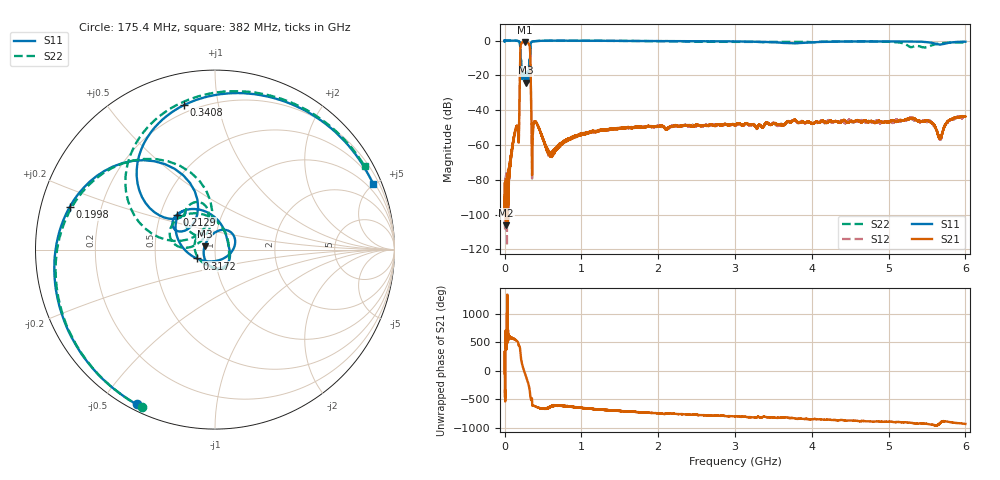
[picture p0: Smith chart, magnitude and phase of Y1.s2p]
!Keysight Technologies,N5232A,MY52221221,A.10.65.11
!Date: Thursday, November 09, 2023 14:39:33
!Correction: S11(Full 2 Port(1,4))
!S41(Full 2 Port(1,4))
!S14(Full 2 Port(1,4))
!S44(Full 2 Port(1,4))
!S2P File: Measurements: S11, S41, S14, S44:
# Hz S  RI  R 50
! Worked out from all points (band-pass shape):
!   16001 points, 300 kHz to 6 GHz, reference 50 ohm
!   highest |S21| = -0.94 dB at 262 MHz (marker M1); lowest = -106.2 dB at 17.92 MHz (marker M2)
!   |S21| within 3 dB of the highest: 206.4 MHz to 329.4 MHz (123 MHz wide, 45.9 % of centre)
!   lowest |S11| = -24.3 dB at 273.3 MHz (marker M3), VSWR 1.13, Z = 44.5 + j1.64 ohm
!   |S11| at or under -10 dB: 206 MHz to 331.9 MHz (125.9 MHz wide, 46.8 % of centre)
!   |S22| runs from -22.2 to 0.0 dB; largest |S21 - S12| = 0.0022
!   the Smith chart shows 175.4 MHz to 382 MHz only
!   S11 on the Smith chart (normalised r, x): 175.4 MHz: 0.02, -0.62; 199.8 MHz: 0.09, +0.14; 212.9 MHz: 0.61, +0.26; 317.2 MHz: 0.81, -0.08; 340.8 MHz: 0.16, +0.80; 382 MHz: 0.61, +4.95
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300000  1.004 -0.00731  5.71e-05 -5.35e-05  3.24e-05 7.01e-06  1.002 -0.0072
1.792412e7  0.9906 -0.133  2.49e-08 4.88e-06  -8.13e-06 -1.72e-05  0.9906 -0.1309
1.086696e8  0.6161 -0.781  -0.000926 -0.00061  -0.000994 -0.000492  0.6305 -0.7709
1.754162e8  -0.4349 -0.8627  -0.00166 0.00147  -0.00174 0.00153  -0.4061 -0.8797
1.9979e8  -0.8096 0.2377  0.0819 0.0818  0.0819 0.0816  -0.7913 0.2473
2.129144e8  -0.2112 0.1954  -0.5439 -0.5433  -0.5434 -0.5435  -0.2351 0.1437
2.305385e8  0.0738 0.0291  -0.2171 0.8498  -0.2173 0.8493  0.0779 0.0046
2.620369e8  -0.0492 -0.068  0.7637 -0.4717  0.7629 -0.4717  0.00628 -0.1071
2.732864e8  -0.0581 0.0184  0.2434 -0.8607  0.2437 -0.86  -0.0247 -0.0936
3.171592e8  -0.1022 -0.0491  -0.00435 0.7967  -0.00382 0.7967  -0.1355 0.0967
3.40783e8  -0.1722 0.8054  -0.0524 -0.0537  -0.0523 -0.0538  -0.3108 0.7425
3.820309e8  0.8809 0.3653  -0.00121 0.00405  -0.00118 0.00411  0.834 0.4635
4.187791e8  0.9697 -0.0672  0.000554 0.00413  0.000571 0.00405  0.9703 0.0288
5.856457e8  0.5238 -0.8398  9.27e-05 0.000515  0.000113 0.000543  0.5965 -0.7904
1.000375e9  -0.4341 -0.8789  0.000793 0.00201  0.00068 0.00192  -0.3419 -0.9246
2.00045e9  -0.9638 -0.0109  0.00305 -0.0014  0.00318 -0.00157  -0.95 -0.1292
3.00015e9  -0.767 0.5353  0.000631 -0.00364  0.000428 -0.00371  -0.8364 0.3724
4.000225e9  -0.5289 0.7142  -0.00272 -0.00306  -0.00276 -0.00329  -0.5767 0.6944
5.0003e9  -0.1583 0.9292  -0.00451 -0.000332  -0.00485 -0.000173  -0.134 0.9114
5.535398e9  0.1271 0.8721  -0.00345 0.0031  -0.00377 0.00309  -0.156 0.671
5.671516e9  0.0803 0.762  -0.00151 0.000457  -0.00133 0.000464  -0.1208 0.8256
6e9  0.1779 0.9055  -0.00546 0.00359  -0.00586 0.00364  0.127 0.8648
